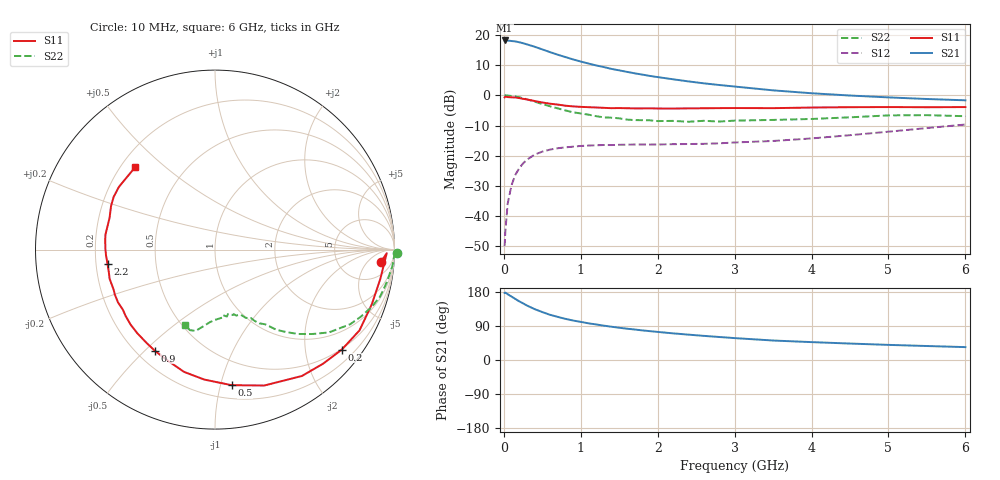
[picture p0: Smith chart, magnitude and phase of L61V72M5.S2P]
!  INFINEON TECHNOLOGIES Small Signal Semiconductors
! BFR380L3 , Si-NPN RF-Transistor in TSLP-3-1
!  Vce=1.75 V,  Ic=2.5 mA
! Common Emitter S-Parameters:  07. March 2005
#  GHz  S  MA  R  50
! f  S11  S21  S12  S22
! GHz  Mag  Ang  Mag  Ang  Mag  Ang  Mag  Ang
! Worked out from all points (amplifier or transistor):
!   36 points, 10 MHz to 6 GHz, reference 50 ohm
!   highest |S21| = 18.1 dB at 10 MHz (marker M1)
!   |S21| within 3 dB of that: start of sweep to 504.9 MHz
!   unconditionally stable (mu >= 1): 2.701 GHz to 4.721 GHz
!   at 250 MHz: K = 0.10, MSG = 19.9 dB, |S12| = -22.5 dB
!   at 1.4 GHz: K = 0.60, MSG = 12.6 dB, |S12| = -16.5 dB
!   at 6 GHz: K = 0.92, MSG = 4.0 dB, |S12| = -9.7 dB
!   S11 on the Smith chart (normalised r, x): 10 MHz: 13, -13; 200 MHz: 0.48, -2.81; 500 MHz: 0.30, -1.08; 900 MHz: 0.27, -0.54; 2.2 GHz: 0.25, -0.06; 6 GHz: 0.26, +0.40
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0.01  0.9257 -4.4  8.078 177.1  0.0032 85.0  1.014 -1.1
0.02  0.9571 -1.2  8.03 177.8  0.0057 87.3  0.9985 -2.3
0.05  0.9355 -10.0  8.048 173.6  0.0162 86.7  0.9921 -5.4
0.1  0.9253 -19.2  7.909 167.4  0.0327 79.9  0.9749 -10.6
0.15  0.9224 -29.2  7.792 161.0  0.0485 74.6  0.9564 -15.9
0.2  0.8997 -38.3  7.543 154.8  0.0622 69.6  0.9291 -20.2
0.3  0.8545 -55.5  6.964 143.8  0.086 60.8  0.8603 -28.9
0.4  0.8054 -70.1  6.361 134.3  0.1045 53.8  0.7849 -36.0
0.5  0.7611 -83.0  5.748 126.5  0.1171 48.2  0.717 -41.0
0.6  0.7267 -94.7  5.181 119.3  0.1265 43.6  0.659 -45.5
0.7  0.7028 -104.2  4.7 113.8  0.1332 40.6  0.6082 -49.1
0.8  0.6736 -112.6  4.293 108.6  0.1379 37.7  0.5633 -52.5
0.9  0.6558 -120.8  3.924 104.2  0.1415 35.5  0.5236 -54.7
1.1  0.6362 -132.7  3.355 96.8  0.1478 32.9  0.4791 -59.0
1.3  0.6205 -143.3  2.932 90.6  0.1508 31.4  0.4317 -62.2
1.6  0.6117 -155.8  2.442 82.6  0.1526 30.9  0.3969 -67.7
2.2  0.604 -172.2  1.841 70.3  0.1556 34.0  0.3776 -74.7
2.8  0.614 175.0  1.481 60.7  0.1607 40.5  0.368 -83.1
3.5  0.6134 163.3  1.208 51.4  0.1758 47.7  0.3919 -90.2
4.5  0.6363 152.6  0.992 43.4  0.2192 58.0  0.4325 -98.7
5.5  0.6354 140.8  0.869 36.9  0.2872 62.2  0.4699 -107.3
6  0.6392 134.0  0.827 34.0  0.3288 62.1  0.4514 -112.0
